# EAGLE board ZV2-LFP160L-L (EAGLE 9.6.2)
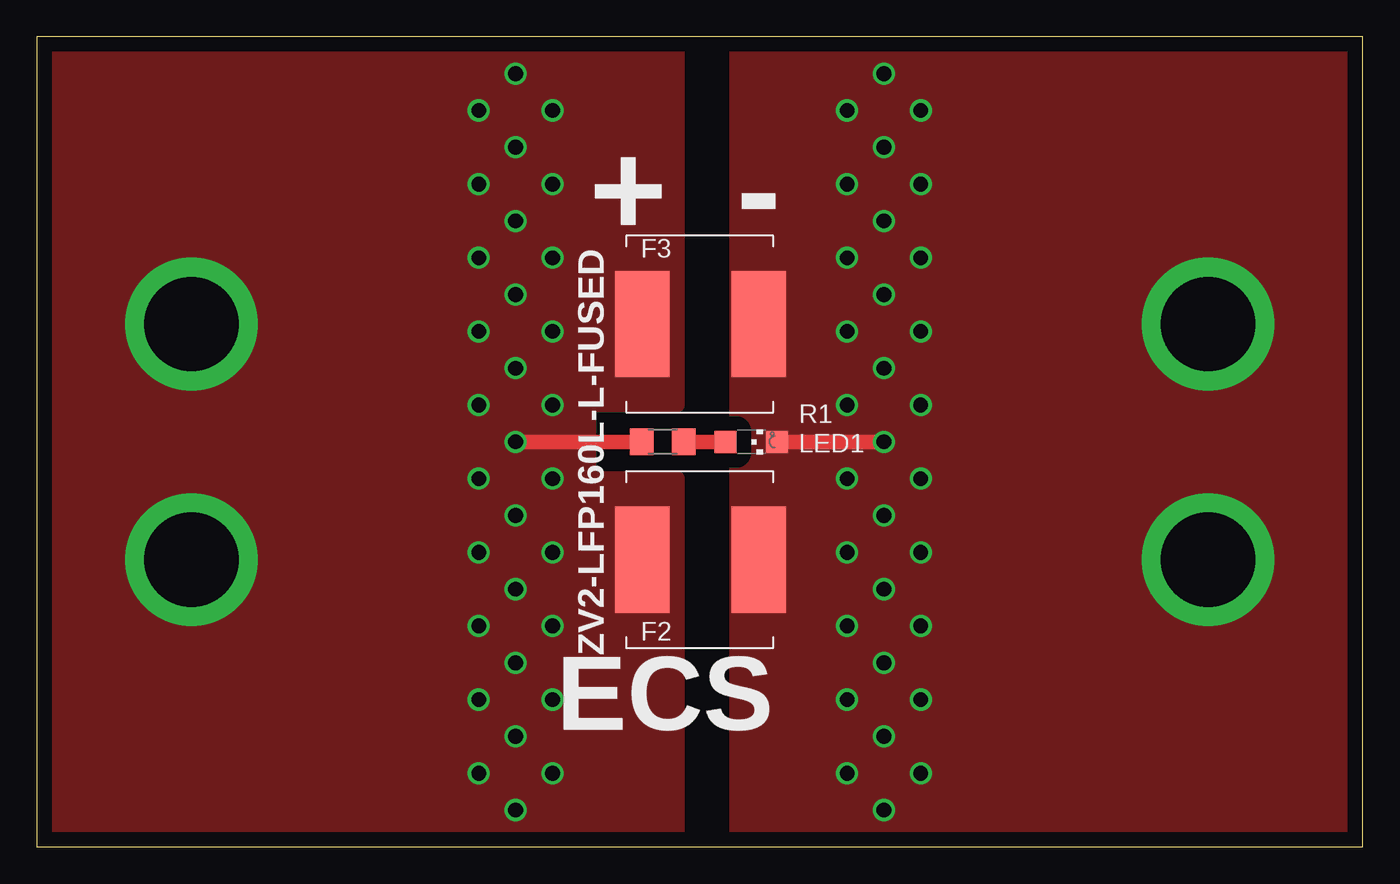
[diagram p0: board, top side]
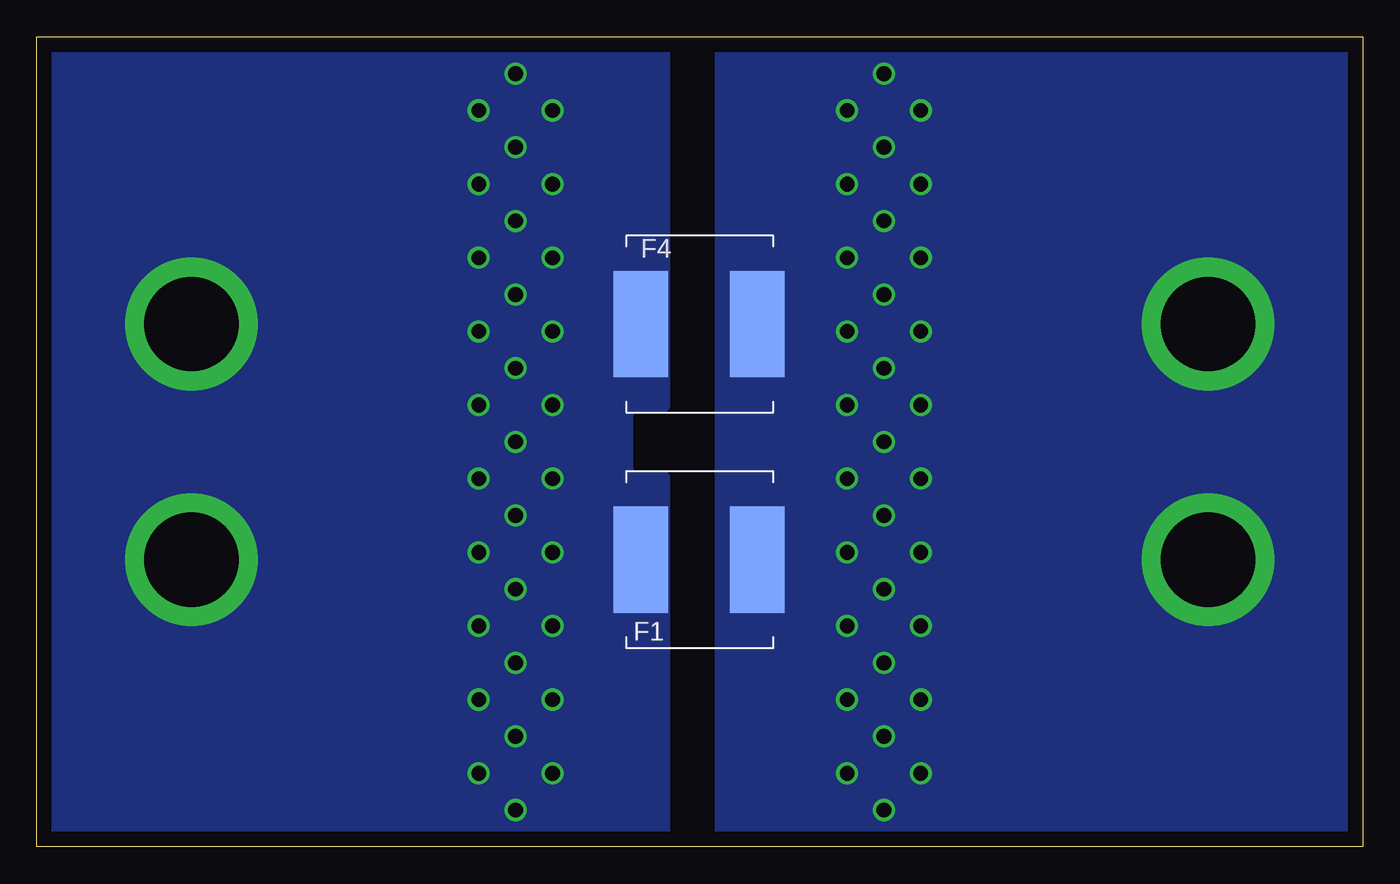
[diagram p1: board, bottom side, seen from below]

Size 90 x 55 mm. Coordinates in mm from the lower left corner, seen from the top.
Outline: 0,0 90,0 90,55 0,55 0,0
Copper layers (1*16): Top 0.035mm / dielectric 1.5mm / Bottom 0.035mm
Design rules "default": minimum track width 6mil, minimum drill 0.35mm, track to track 6mil, track to pad 6mil, pad to pad 6mil, via to via 6mil, smd to smd 6mil, copper to edge 40mil, drill to drill 6mil, minimum pad ring 10mil, minimum via ring 8mil, stop-mask expansion 4mil, vias tented up to drill 0mil, thermal gap 10mil

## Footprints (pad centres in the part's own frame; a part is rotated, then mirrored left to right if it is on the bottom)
UHP = smd 3.7 x 7.2: 1 -3.9,0; 2 4,0
6,4 = drill 6.4 pad 9: B6,4 0,0
CHIPLED_1206 = smd 1.5 x 1.5: A 0,-1.75; C 0,1.75
R1206 = smd 1.6 x 1.803: 1 -1.422,0; 2 1.422,0

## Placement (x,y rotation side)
F1  [UHP]  45,19.5 180 bottom
F2  [UHP]  45,19.5 0 top
F3  [UHP]  45,35.5 0 top
F4  [UHP]  45,35.5 180 bottom
H1  MOUNT-PAD-ROUND  [6,4]  10.5,35.5 0 top
H2  MOUNT-PAD-ROUND  [6,4]  10.5,19.5 0 top
H3  MOUNT-PAD-ROUND  [6,4]  79.5,19.5 0 top
H4  MOUNT-PAD-ROUND  [6,4]  79.5,35.5 0 top
LED1  [CHIPLED_1206]  48.5,27.5 270 top
R1  470R  [R1206]  42.5,27.5 0 top

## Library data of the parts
F1-F4 = schurter_fuse
H1-H4 = holes
LED1 = led
R1 = rcl; SPICEPREFIX: R

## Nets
1: F1.1 F2.1 F3.1 F4.1 H1.B6,4 H2.B6,4 R1.1
2: F1.2 F2.2 F3.2 F4.2 H3.B6,4 H4.B6,4 LED1.C
N$2: LED1.A R1.2

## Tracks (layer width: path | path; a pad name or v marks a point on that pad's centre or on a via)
1  (via drill 1)
  Top 1: R1.1 v32.5,27.5
  other vias: 32.5,42.5 30,40 35,40 32.5,37.5 30,35 35,35 32.5,32.5 30,30 35,30 30,25 35,25 32.5,22.5 30,20 35,20 32.5,17.5 30,15 35,15 32.5,12.5 35,45 30,45 32.5,47.5 35,50 30,50 32.5,52.5 30,10 35,10 32.5,7.5 35,5 32.5,2.5 30,5
  pour Top (isolate 1, no thermals): 0,55 43.5,55 43.5,30 37.5,30 37.5,25 43.5,25 43.5,0 0,0
  pour Bottom (no thermals): 0,55 43.5,55 43.5,0 0,0
2  (via drill 1)
  Top 1: LED1.C v57.5,27.5
  other vias: 57.5,42.5 55,40 60,40 57.5,37.5 55,35 60,35 57.5,32.5 55,30 60,30 55,25 60,25 57.5,22.5 60,20 55,20 57.5,17.5 55,15 60,15 57.5,12.5 55,10 57.5,7.5 60,10 60,5 55,5 57.5,2.5 60,45 55,45 57.5,47.5 60,50 55,50 57.5,52.5
  pour Top (isolate 1, no thermals): 47.5,55 90,55 90,0 47.5,0
  pour Bottom (no thermals): 47.5,55 90,55 90,0 47.5,0 47.5,25 50,25 50,30 47.5,30
N$2
  Top 1: R1.2 LED1.A

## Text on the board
tPlace: + | - | ZV2-LFP160L-L-FUSED | ECS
